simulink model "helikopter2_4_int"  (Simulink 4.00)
settings: Solver=ode1  SolverMode=SingleTasking  StartTime=0.0  StopTime=999999  FixedStep=0.005  MaxStep=10  RelTol=1e-3  AbsTol=1e-3
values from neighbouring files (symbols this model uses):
  K = place(a,b,p)    [init3.m]
undefined symbols (not defined in the file or in its folder): simget
libraries: qctools x7

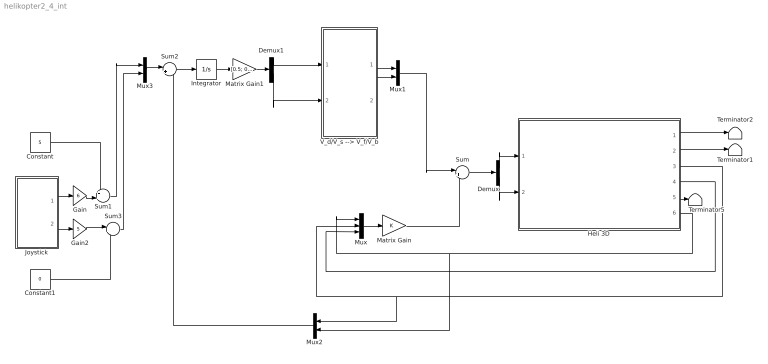
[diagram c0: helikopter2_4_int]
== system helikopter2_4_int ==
  Constant : Constant  Value=5
  Constant1 : Constant  Value=0
  Demux : Demux  Outputs=2  BusSelectionMode=off
  Demux1 : Demux  Outputs=2  BusSelectionMode=off
  Gain : Gain  Gain=6  Multiplication=Element-wise(K.*u)  SaturateOnIntegerOverflow=on
  Gain2 : Gain  Gain=5  Multiplication=Element-wise(K.*u)  SaturateOnIntegerOverflow=on
  Heli 3D : Subsystem
  Integrator : Integrator  ExternalReset=none  InitialConditionSource=internal  InitialCondition=0  LimitOutput=off  UpperSaturationLimit=inf  LowerSaturationLimit=-inf  ShowSaturationPort=off  ShowStatePort=off  AbsoluteTolerance=auto
  Joystick : Subsystem
  Matrix Gain : Gain  Gain=K  Multiplication=Matrix(K*u)  SaturateOnIntegerOverflow=on
  Matrix Gain1 : Gain  Gain=[0.5; 0.5]  Multiplication=Element-wise(K.*u)  SaturateOnIntegerOverflow=on
  Mux : Mux  Inputs=3
  Mux1 : Mux  Inputs=2
  Mux2 : Mux  Orientation=left  Inputs=2
  Mux3 : Mux  Inputs=2
  Sum : Sum  Inputs=|+-  SaturateOnIntegerOverflow=on
  Sum1 : Sum  Inputs=++|  SaturateOnIntegerOverflow=on
  Sum2 : Sum  Inputs=|+-  SaturateOnIntegerOverflow=on
  Sum3 : Sum  Inputs=|++  SaturateOnIntegerOverflow=on
  Terminator1 : Terminator
  Terminator2 : Terminator
  Terminator5 : Terminator
  V_d/V_s --> V_f/V_b : Subsystem
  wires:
  Joystick/1(X Volt) -> Gain/1
  Heli 3D/1("Vandring, (grader)") -> Terminator2/1
  Joystick/2(Y Volt) -> Gain2/1
  Mux/1 -> Matrix Gain/1
  Demux/1 -> Heli 3D/1("V_f, motor foran")
  Demux/2 -> Heli 3D/2("V_b, motor bak")
  V_d/V_s --> V_f/V_b/1(V_f) -> Mux1/1
  V_d/V_s --> V_f/V_b/2(V_b) -> Mux1/2
  Heli 3D/2("Vandringsrate, (grader/sek)") -> Terminator1/1
  Sum/1 -> Demux/1
  Mux1/1 -> Sum/1
  Matrix Gain/1 -> Sum/2
  Mux2/1 -> Sum2/2
  Mux3/1 -> Sum2/1
  Demux1/1 -> V_d/V_s --> V_f/V_b/1(V_d)
  Demux1/2 -> V_d/V_s --> V_f/V_b/2(V_s)
  Sum2/1 -> Integrator/1
  Matrix Gain1/1 -> Demux1/1
  Integrator/1 -> Matrix Gain1/1
  Heli 3D/5("Elevasjon, (grader)") -> Terminator5/1
  Heli 3D/3("Pitch, (grader)") -> Mux/2, Mux2/1
  Heli 3D/4("Pitchrate, (grader/sek)") -> Mux/3
  Heli 3D/6(Elevasjonsrate (grader/sek)) -> Mux/1, Mux2/2
  Gain2/1 -> Sum3/1
  Constant1/1 -> Sum3/2
  Sum3/1 -> Mux3/2
  Gain/1 -> Sum1/2
  Constant/1 -> Sum1/1
  Sum1/1 -> Mux3/1

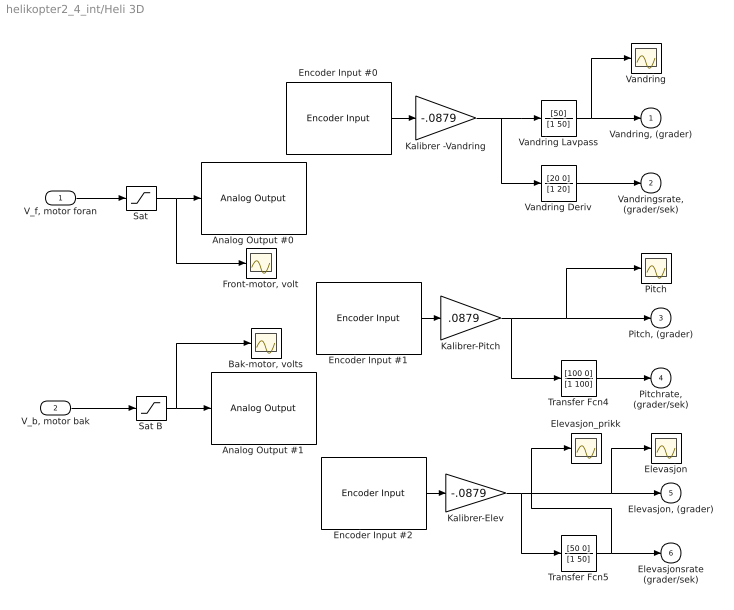
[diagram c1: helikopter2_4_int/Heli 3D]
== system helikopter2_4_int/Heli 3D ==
  "V_f, motor foran" : Inport  Port=1  LatchInput=off
  "V_b, motor bak" : Inport  Port=2  LatchInput=off
  Analog Output #0 : qctools/Quanser Consulting MQ3 Series/Analog Output  baseAddr=0x320  channels=0  initialOutputs=0  finalOutputs=0  sampleTime=-1  simulationOutput=off
  Analog Output #1 : qctools/Quanser Consulting MQ3 Series/Analog Output  baseAddr=0x320  channels=1  initialOutputs=0  finalOutputs=0  sampleTime=-1  simulationOutput=off
  "Bak-motor, volts" : Scope
  Elevasjon : Scope
  Elevasjon_prikk : Scope
  Encoder Input #0 : qctools/Quanser Consulting MQ3 Series/Encoder Input  baseAddr=0x320  channels=0  initialValues=0  sampleTime=simget(bdroot,'FixedStep')  simulationInput=off
  Encoder Input #1 : qctools/Quanser Consulting MQ3 Series/Encoder Input  baseAddr=0x320  channels=1  initialValues=0  sampleTime=simget(bdroot,'FixedStep')  simulationInput=off
  Encoder Input #2 : qctools/Quanser Consulting MQ3 Series/Encoder Input  baseAddr=0x320  channels=2  initialValues=0  sampleTime=simget(bdroot,'FixedStep')  simulationInput=off
  "Front-motor, volt" : Scope
  Kalibrer -Vandring : Gain  Gain=-.0879  Multiplication=Element-wise(K.*u)  SaturateOnIntegerOverflow=on
  Kalibrer-Elev : Gain  Gain=-.0879  Multiplication=Element-wise(K.*u)  SaturateOnIntegerOverflow=on
  Kalibrer-Pitch : Gain  Gain=.0879  Multiplication=Element-wise(K.*u)  SaturateOnIntegerOverflow=on
  Pitch : Scope
  Sat : Saturate  UpperLimit=5  LowerLimit=-5  LinearizeAsGain=on
  Sat B : Saturate  UpperLimit=5  LowerLimit=-5  LinearizeAsGain=on
  Transfer Fcn4 : TransferFcn  Numerator=[100 0]  Denominator=[1 100]  AbsoluteTolerance=auto  Realization=auto
  Transfer Fcn5 : TransferFcn  Numerator=[50 0]  Denominator=[1 50]  AbsoluteTolerance=auto  Realization=auto
  Vandring : Scope
  Vandring Deriv : TransferFcn  Numerator=[20 0]  Denominator=[1 20]  AbsoluteTolerance=auto  Realization=auto
  Vandring Lavpass : TransferFcn  Numerator=[50]  Denominator=[1 50]  AbsoluteTolerance=auto  Realization=auto
  "Vandring, (grader)" : Outport  Port=1  InitialOutput=0
  "Vandringsrate, (grader/sek)" : Outport  Port=2  InitialOutput=0
  "Pitch, (grader)" : Outport  Port=3  InitialOutput=0
  "Pitchrate, (grader/sek)" : Outport  Port=4  InitialOutput=0
  "Elevasjon, (grader)" : Outport  Port=5  InitialOutput=0
  Elevasjonsrate (grader/sek) : Outport  Port=6  InitialOutput=0
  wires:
  Vandring Deriv/1 -> "Vandringsrate, (grader/sek)"/1
  Vandring Lavpass/1 -> Vandring/1, "Vandring, (grader)"/1
  Encoder Input #0/1 -> Kalibrer -Vandring/1
  Kalibrer -Vandring/1 -> Vandring Deriv/1, Vandring Lavpass/1
  Encoder Input #1/1 -> Kalibrer-Pitch/1
  Kalibrer-Pitch/1 -> Pitch/1, "Pitch, (grader)"/1, Transfer Fcn4/1
  Transfer Fcn4/1 -> "Pitchrate, (grader/sek)"/1
  Encoder Input #2/1 -> Kalibrer-Elev/1
  Kalibrer-Elev/1 -> Transfer Fcn5/1, Elevasjon/1, "Elevasjon, (grader)"/1
  Transfer Fcn5/1 -> Elevasjonsrate (grader/sek)/1, Elevasjon_prikk/1
  Sat/1 -> "Front-motor, volt"/1, Analog Output #0/1
  Sat B/1 -> "Bak-motor, volts"/1, Analog Output #1/1
  "V_f, motor foran"/1 -> Sat/1
  "V_b, motor bak"/1 -> Sat B/1

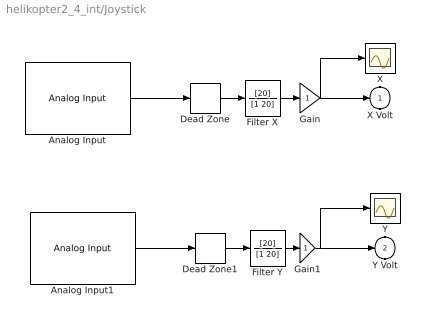
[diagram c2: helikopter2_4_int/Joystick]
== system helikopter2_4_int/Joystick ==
  Analog Input : qctools/Quanser Consulting MQ3 Series/Analog Input  baseAddr=0x320  channels=2  sampleTime=simget(bdroot,'FixedStep')  simulationInput=off
  Analog Input1 : qctools/Quanser Consulting MQ3 Series/Analog Input  baseAddr=0x320  channels=3  sampleTime=simget(bdroot,'FixedStep')  simulationInput=off
  Dead Zone : DeadZone  LowerValue=-0.5  UpperValue=0.5  SaturateOnIntegerOverflow=on  LinearizeAsGain=on
  Dead Zone1 : DeadZone  LowerValue=-0.5  UpperValue=0.5  SaturateOnIntegerOverflow=on  LinearizeAsGain=on
  Filter X : TransferFcn  Numerator=[20]  Denominator=[1 20]  AbsoluteTolerance=auto  Realization=auto
  Filter Y : TransferFcn  Numerator=[20]  Denominator=[1 20]  AbsoluteTolerance=auto  Realization=auto
  Gain : Gain  Gain=1  Multiplication=Element-wise(K.*u)  SaturateOnIntegerOverflow=on
  Gain1 : Gain  Gain=1  Multiplication=Element-wise(K.*u)  SaturateOnIntegerOverflow=on
  X : Scope
  Y : Scope
  X Volt : Outport  Port=1  InitialOutput=0
  Y Volt : Outport  Port=2  InitialOutput=0
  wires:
  Dead Zone/1 -> Filter X/1
  Analog Input1/1 -> Dead Zone1/1
  Dead Zone1/1 -> Filter Y/1
  Filter Y/1 -> Gain1/1
  Filter X/1 -> Gain/1
  Analog Input/1 -> Dead Zone/1
  Gain/1 -> X Volt/1, X/1
  Gain1/1 -> Y Volt/1, Y/1

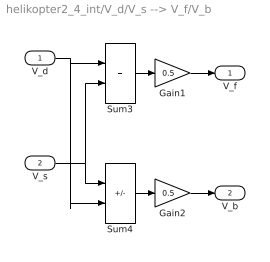
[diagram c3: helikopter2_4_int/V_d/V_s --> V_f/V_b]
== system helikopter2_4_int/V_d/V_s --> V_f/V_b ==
  V_d : Inport  Port=1  LatchInput=off
  V_s : Inport  Port=2  LatchInput=off
  Gain1 : Gain  Gain=0.5  Multiplication=Element-wise(K.*u)  SaturateOnIntegerOverflow=on
  Gain2 : Gain  Gain=0.5  Multiplication=Element-wise(K.*u)  SaturateOnIntegerOverflow=on
  Sum3 : Sum  Inputs=++  SaturateOnIntegerOverflow=on
  Sum4 : Sum  Inputs=+-  SaturateOnIntegerOverflow=on
  V_f : Outport  Port=1  InitialOutput=0
  V_b : Outport  Port=2  InitialOutput=0
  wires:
  V_s/1 -> Sum4/1, Sum3/2
  Sum3/1 -> Gain1/1
  Sum4/1 -> Gain2/1
  V_d/1 -> Sum3/1, Sum4/2
  Gain1/1 -> V_f/1
  Gain2/1 -> V_b/1
